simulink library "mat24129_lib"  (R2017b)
settings: Solver=VariableStepAuto  StartTime=0.0  StopTime=10.0  RelTol=1e-3
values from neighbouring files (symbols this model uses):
  beta = 0.1    [lh2t4_DOC.m]
  c = 1000    [lh2t4_DOC.m]
  g = 9.8    [lh2t4_DOC.m]
  H = 2000    [lh2t4_DOC.m]
  h0 = 1    [lh2t4_DOC.m]
  m0 = 1000    [lh2t4_DOC.m]
  m_start = 500    [lh2t4_DOC.m]
  v0 = 1    [lh2t4_DOC.m]
libraries: mat24129_lib x2

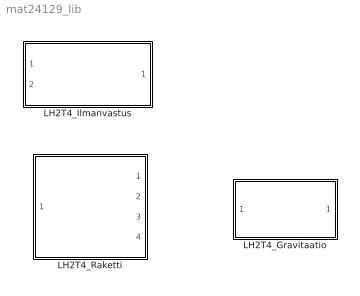
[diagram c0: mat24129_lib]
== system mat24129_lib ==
  LH2T4_Gravitaatio : Subsystem
  LH2T4_Ilmanvastus : Subsystem
  LH2T4_Raketti : Subsystem

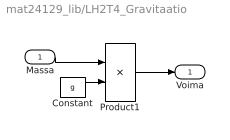
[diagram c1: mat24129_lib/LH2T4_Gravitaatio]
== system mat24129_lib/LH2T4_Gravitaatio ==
  Massa : Inport
  Constant : Constant  Value=g
  Product1 : Product
  Voima : Outport
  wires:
  Massa/1 -> Product1/1
  Product1/1 -> Voima/1
  Constant/1 -> Product1/2

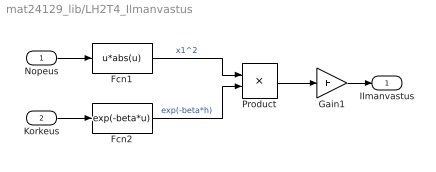
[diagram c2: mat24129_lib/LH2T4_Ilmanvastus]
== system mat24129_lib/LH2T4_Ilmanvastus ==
  Nopeus : Inport
  Korkeus : Inport  Port=2
  Fcn1 : Fcn  Expr=u*abs(u)
  Fcn2 : Fcn  Expr=exp(-beta*u)
  Gain1 : Gain  Gain=H
  Product : Product
  Ilmanvastus : Outport
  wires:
  Fcn1/1 -> Product/1  "x1^2"
  Fcn2/1 -> Product/2  "exp(-beta*h)"
  Product/1 -> Gain1/1
  Nopeus/1 -> Fcn1/1
  Korkeus/1 -> Fcn2/1
  Gain1/1 -> Ilmanvastus/1

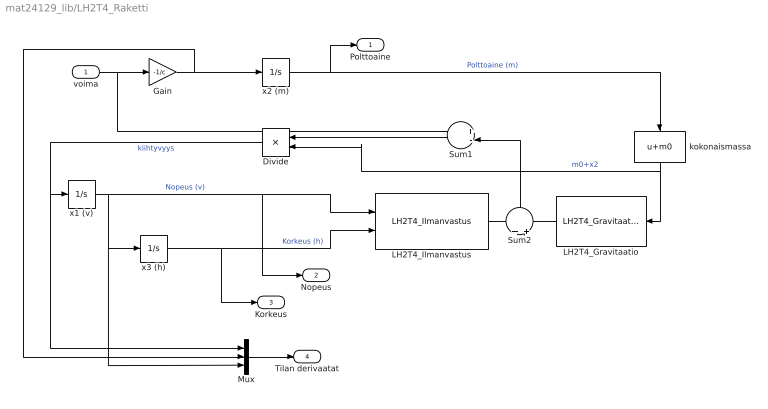
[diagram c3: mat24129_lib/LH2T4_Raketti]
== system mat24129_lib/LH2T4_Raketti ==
  voima : Inport
  Divide : Product  Inputs=*/
  Gain : Gain  Gain=-1/c
  LH2T4_Gravitaatio : mat24129_lib/LH2T4_Gravitaatio
  LH2T4_Ilmanvastus : mat24129_lib/LH2T4_Ilmanvastus
  Mux : Mux  Inputs=3
  Sum1 : Sum  Inputs=+-|
  Sum2 : Sum  Inputs=+|+
  kokonaismassa : Fcn  Expr=u+m0
  x1 (v) : Integrator  InitialCondition=v0  LowerSaturationLimit=-10000
  x2 (m) : Integrator  InitialCondition=m_start
  x3 (h) : Integrator  InitialCondition=h0  LimitOutput=on  LowerSaturationLimit=-eps
  Polttoaine : Outport
  Nopeus : Outport  Port=2
  Korkeus : Outport  Port=3
  Tilan derivaatat : Outport  Port=4
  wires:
  x1 (v)/1 -> Nopeus/1, LH2T4_Ilmanvastus/1, x3 (h)/1, Mux/3  "Nopeus (v)"
  x2 (m)/1 -> Polttoaine/1, kokonaismassa/1  "Polttoaine (m)"
  x3 (h)/1 -> Korkeus/1, LH2T4_Ilmanvastus/2  "Korkeus (h)"
  Gain/1 -> x2 (m)/1, Mux/2
  Divide/1 -> Mux/1, x1 (v)/1  "kiihtyvyys"
  voima/1 -> Gain/1, Sum1/1
  Sum2/1 -> Sum1/2
  Sum1/1 -> Divide/1
  kokonaismassa/1 -> Divide/2, LH2T4_Gravitaatio/1  "m0+x2"
  LH2T4_Gravitaatio/1 -> Sum2/2
  LH2T4_Ilmanvastus/1 -> Sum2/1
  Mux/1 -> Tilan derivaatat/1
